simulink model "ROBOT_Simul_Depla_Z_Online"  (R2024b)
settings: Solver=ode15s  StartTime=0.0  StopTime=0.2  RelTol=1e-3  EnableMultiTasking=on
undefined symbols (not defined in the file): BATI1_Défaut_sldprt, BATI2_Défaut_sldprt, BATI3_Défaut_sldprt, BIELLE_Défaut_sldprt, BRAS_Défaut_sldprt, deg, Drive, EFFECTEUR_Défaut_sldprt, Fichiers, Fichiers_Matlab_sujetB, JOINT_Défaut_sldprt, kg, m, MANETTE_Défaut_sldprt, MATLAB, Matlab, mm, N, PIED_Défaut_sldprt, rad, s, STL, X, Y, Z
libraries: sm_lib x139, fl_lib x42, nesl_utility x19, slpidlib x3
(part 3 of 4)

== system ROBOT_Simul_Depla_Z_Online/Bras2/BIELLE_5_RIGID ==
  ReferenceFrame : sm_lib/Frames and Transforms/Reference Frame
  Solid : sm_lib/Body Elements/File Solid  ExtGeomFileName=/MATLAB Drive/Fichiers_Matlab_sujetB/Fichiers Matlab/STL/BIELLE_Défaut_sldprt.STL  UnitType=Custom  ExtGeomFileUnits=mm  StepReaderType=HEX  ExportConvexHullGeometry=off  InertiaType=Custom  BasedOnType=Density  Density=1000  DensityUnits=kg/(m^3)  Mass=0.008350539405564527  MassUnits=kg  CenterOfMass=[0 1.3968069938607398e-07 -5.4963035279888423e-06]  CenterOfMassUnits=mm  MomentsOfInertia=[9.7237898508136684 9.7147278737202658 0.035523108889582884]  MomentsOfInertiaUnits=kg*mm^2  ProductsOfInertia=[0 -4.4011490170351759e-08 -8.1673382975267321e-07]  ProductsOfInertiaUnits=kg*mm^2  GraphicType=FromGeometry  MarkerShape=Sphere  MarkerSize=10  GraphicVisPropType=SimpleVisualProperties  GraphicDiffuseColor=[0.69803921568627447 0.69803921568627447 0.69803921568627447]  GraphicOpacity=1  GraphicSpecularColor=[0.5 0.5 0.5 1.0]  GraphicAmbientColor=[0.15 0.15 0.15 1.0]  GraphicEmissiveColor=[0.0 0.0 0.0 1.0]  GraphicShininess=75  DoExposeReferenceFrame=on  SerializedFrames=<Frames/>
  Transform : sm_lib/Frames and Transforms/Rigid Transform  RotationMethod=ArbitraryAxis  FollAlignAxisA=+X  BaseAlignAxisA=+Y  FollAlignAxisB=+Y  BaseAlignAxisB=+Z  RotationStandardAxis=+Z  RotationAngle=2.0943951023931953  RotationAngleUnits=rad  RotationArbitraryAxis=[0.57735026918962584 -0.57735026918962584 0.57735026918962584]  RotationSequenceAxes=FollowerAxes  RotationSequence=XYX  RotationSequenceAngles=[0 0 0]  RotationSequenceAnglesUnits=deg  RotationMatrix=[1 0 0; 0 1 0; 0 0 1]  Quaternion=[1 0 0 0]  TranslationMethod=Cartesian  TranslationCartesianOffset=[0 4.9999999999999973 -51.250000000000007]  TranslationCartesianOffsetUnits=mm  TranslationStandardAxis=+Z  TranslationStandardOffset=0  TranslationStandardOffsetUnits=mm  TranslationROffset=0  TranslationROffsetUnits=m  TranslationThetaOffset=0  TranslationThetaOffsetUnits=deg  TranslationZOffset=0  TranslationZOffsetUnits=m
  Transform1 : sm_lib/Frames and Transforms/Rigid Transform  RotationMethod=ArbitraryAxis  FollAlignAxisA=+X  BaseAlignAxisA=+Y  FollAlignAxisB=+Y  BaseAlignAxisB=+Z  RotationStandardAxis=+Z  RotationAngle=2.0943951023931953  RotationAngleUnits=rad  RotationArbitraryAxis=[0.57735026918962584 -0.57735026918962584 0.57735026918962584]  RotationSequenceAxes=FollowerAxes  RotationSequence=XYX  RotationSequenceAngles=[0 0 0]  RotationSequenceAnglesUnits=deg  RotationMatrix=[1 0 0; 0 1 0; 0 0 1]  Quaternion=[1 0 0 0]  TranslationMethod=Cartesian  TranslationCartesianOffset=[0 5.0000000000000044 51.249999999999993]  TranslationCartesianOffsetUnits=mm  TranslationStandardAxis=+Z  TranslationStandardOffset=0  TranslationStandardOffsetUnits=mm  TranslationROffset=0  TranslationROffsetUnits=m  TranslationThetaOffset=0  TranslationThetaOffsetUnits=deg  TranslationZOffset=0  TranslationZOffsetUnits=m
  F : PMIOPort  Side=Left
  F1 : PMIOPort  Port=2  Side=Right
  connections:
  Solid/RConn1 -- ReferenceFrame/RConn1 -- Transform/LConn1 -- Transform1/LConn1
  Transform/RConn1 -- F/RConn1
  Transform1/RConn1 -- F1/RConn1

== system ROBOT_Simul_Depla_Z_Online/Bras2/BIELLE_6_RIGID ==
  ReferenceFrame : sm_lib/Frames and Transforms/Reference Frame
  Solid : sm_lib/Body Elements/File Solid  ExtGeomFileName=/MATLAB Drive/Fichiers_Matlab_sujetB/Fichiers Matlab/STL/BIELLE_Défaut_sldprt.STL  UnitType=Custom  ExtGeomFileUnits=mm  StepReaderType=HEX  ExportConvexHullGeometry=off  InertiaType=Custom  BasedOnType=Density  Density=1000  DensityUnits=kg/(m^3)  Mass=0.008350539405564527  MassUnits=kg  CenterOfMass=[0 1.3968069938607398e-07 -5.4963035279888423e-06]  CenterOfMassUnits=mm  MomentsOfInertia=[9.7237898508136684 9.7147278737202658 0.035523108889582884]  MomentsOfInertiaUnits=kg*mm^2  ProductsOfInertia=[0 -4.4011490170351759e-08 -8.1673382975267321e-07]  ProductsOfInertiaUnits=kg*mm^2  GraphicType=FromGeometry  MarkerShape=Sphere  MarkerSize=10  GraphicVisPropType=SimpleVisualProperties  GraphicDiffuseColor=[0.69803921568627447 0.69803921568627447 0.69803921568627447]  GraphicOpacity=1  GraphicSpecularColor=[0.5 0.5 0.5 1.0]  GraphicAmbientColor=[0.15 0.15 0.15 1.0]  GraphicEmissiveColor=[0.0 0.0 0.0 1.0]  GraphicShininess=75  DoExposeReferenceFrame=on  SerializedFrames=<Frames/>
  Transform : sm_lib/Frames and Transforms/Rigid Transform  RotationMethod=ArbitraryAxis  FollAlignAxisA=+X  BaseAlignAxisA=+Y  FollAlignAxisB=+Y  BaseAlignAxisB=+Z  RotationStandardAxis=+Z  RotationAngle=2.0943951023931953  RotationAngleUnits=rad  RotationArbitraryAxis=[0.57735026918962584 -0.57735026918962584 0.57735026918962584]  RotationSequenceAxes=FollowerAxes  RotationSequence=XYX  RotationSequenceAngles=[0 0 0]  RotationSequenceAnglesUnits=deg  RotationMatrix=[1 0 0; 0 1 0; 0 0 1]  Quaternion=[1 0 0 0]  TranslationMethod=Cartesian  TranslationCartesianOffset=[0 4.9999999999999902 -51.249999999999993]  TranslationCartesianOffsetUnits=mm  TranslationStandardAxis=+Z  TranslationStandardOffset=0  TranslationStandardOffsetUnits=mm  TranslationROffset=0  TranslationROffsetUnits=m  TranslationThetaOffset=0  TranslationThetaOffsetUnits=deg  TranslationZOffset=0  TranslationZOffsetUnits=m
  Transform1 : sm_lib/Frames and Transforms/Rigid Transform  RotationMethod=ArbitraryAxis  FollAlignAxisA=+X  BaseAlignAxisA=+Y  FollAlignAxisB=+Y  BaseAlignAxisB=+Z  RotationStandardAxis=+Z  RotationAngle=2.0943951023931953  RotationAngleUnits=rad  RotationArbitraryAxis=[0.57735026918962584 -0.57735026918962584 0.57735026918962584]  RotationSequenceAxes=FollowerAxes  RotationSequence=XYX  RotationSequenceAngles=[0 0 0]  RotationSequenceAnglesUnits=deg  RotationMatrix=[1 0 0; 0 1 0; 0 0 1]  Quaternion=[1 0 0 0]  TranslationMethod=Cartesian  TranslationCartesianOffset=[0 4.9999999999999902 51.25]  TranslationCartesianOffsetUnits=mm  TranslationStandardAxis=+Z  TranslationStandardOffset=0  TranslationStandardOffsetUnits=mm  TranslationROffset=0  TranslationROffsetUnits=m  TranslationThetaOffset=0  TranslationThetaOffsetUnits=deg  TranslationZOffset=0  TranslationZOffsetUnits=m
  F : PMIOPort  Side=Left
  F1 : PMIOPort  Port=2  Side=Right
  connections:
  Solid/RConn1 -- ReferenceFrame/RConn1 -- Transform/LConn1 -- Transform1/LConn1
  Transform/RConn1 -- F/RConn1
  Transform1/RConn1 -- F1/RConn1

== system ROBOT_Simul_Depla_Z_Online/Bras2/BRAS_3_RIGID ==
  BRAS_1_RIGID : Subsystem
  BRAS_3_RIGID : Subsystem
  ReferenceFrame : sm_lib/Frames and Transforms/Reference Frame
  Transform : sm_lib/Frames and Transforms/Rigid Transform  RotationMethod=ArbitraryAxis  FollAlignAxisA=+X  BaseAlignAxisA=+Y  FollAlignAxisB=+Y  BaseAlignAxisB=+Z  RotationStandardAxis=+Z  RotationAngle=3.1415926535897922  RotationAngleUnits=rad  RotationArbitraryAxis=[1 -3.4968219954323673e-31 -7.4654377952851924e-16]  RotationSequenceAxes=FollowerAxes  RotationSequence=XYX  RotationSequenceAngles=[0 0 0]  RotationSequenceAnglesUnits=deg  RotationMatrix=[1 0 0; 0 1 0; 0 0 1]  Quaternion=[1 0 0 0]  TranslationMethod=Cartesian  TranslationCartesianOffset=[-7.3896444519050419e-13 -16.842456388464797 5.0000000000063061]  TranslationCartesianOffsetUnits=mm  TranslationStandardAxis=+Z  TranslationStandardOffset=0  TranslationStandardOffsetUnits=mm  TranslationROffset=0  TranslationROffsetUnits=m  TranslationThetaOffset=0  TranslationThetaOffsetUnits=deg  TranslationZOffset=0  TranslationZOffsetUnits=m
  Transform1 : sm_lib/Frames and Transforms/Rigid Transform  RotationMethod=ArbitraryAxis  FollAlignAxisA=+X  BaseAlignAxisA=+Y  FollAlignAxisB=+Y  BaseAlignAxisB=+Z  RotationStandardAxis=+Z  RotationAngle=3.1415926535897931  RotationAngleUnits=rad  RotationArbitraryAxis=[1 0 0]  RotationSequenceAxes=FollowerAxes  RotationSequence=XYX  RotationSequenceAngles=[0 0 0]  RotationSequenceAnglesUnits=deg  RotationMatrix=[1 0 0; 0 1 0; 0 0 1]  Quaternion=[1 0 0 0]  TranslationMethod=Cartesian  TranslationCartesianOffset=[0 43.157543611535338 10.000000000006285]  TranslationCartesianOffsetUnits=mm  TranslationStandardAxis=+Z  TranslationStandardOffset=0  TranslationStandardOffsetUnits=mm  TranslationROffset=0  TranslationROffsetUnits=m  TranslationThetaOffset=0  TranslationThetaOffsetUnits=deg  TranslationZOffset=0  TranslationZOffsetUnits=m
  Transform2 : sm_lib/Frames and Transforms/Rigid Transform  RotationMethod=None  FollAlignAxisA=+X  BaseAlignAxisA=+Y  FollAlignAxisB=+Y  BaseAlignAxisB=+Z  RotationStandardAxis=+Z  RotationAngle=0  RotationAngleUnits=deg  RotationArbitraryAxis=[0 0 1]  RotationSequenceAxes=FollowerAxes  RotationSequence=XYX  RotationSequenceAngles=[0 0 0]  RotationSequenceAnglesUnits=deg  RotationMatrix=[1 0 0; 0 1 0; 0 0 1]  Quaternion=[1 0 0 0]  TranslationMethod=Cartesian  TranslationCartesianOffset=[0 -16.842456388464662 6.2762295360840881e-12]  TranslationCartesianOffsetUnits=mm  TranslationStandardAxis=+Z  TranslationStandardOffset=0  TranslationStandardOffsetUnits=mm  TranslationROffset=0  TranslationROffsetUnits=m  TranslationThetaOffset=0  TranslationThetaOffsetUnits=deg  TranslationZOffset=0  TranslationZOffsetUnits=m
  Transform3 : sm_lib/Frames and Transforms/Rigid Transform  RotationMethod=ArbitraryAxis  FollAlignAxisA=+X  BaseAlignAxisA=+Y  FollAlignAxisB=+Y  BaseAlignAxisB=+Z  RotationStandardAxis=+Z  RotationAngle=3.1415926535897931  RotationAngleUnits=rad  RotationArbitraryAxis=[0 0 1]  RotationSequenceAxes=FollowerAxes  RotationSequence=XYX  RotationSequenceAngles=[0 0 0]  RotationSequenceAnglesUnits=deg  RotationMatrix=[1 0 0; 0 1 0; 0 0 1]  Quaternion=[1 0 0 0]  TranslationMethod=Cartesian  TranslationCartesianOffset=[0 43.157543611535338 6.2692906421801808e-12]  TranslationCartesianOffsetUnits=mm  TranslationStandardAxis=+Z  TranslationStandardOffset=0  TranslationStandardOffsetUnits=mm  TranslationROffset=0  TranslationROffsetUnits=m  TranslationThetaOffset=0  TranslationThetaOffsetUnits=deg  TranslationZOffset=0  TranslationZOffsetUnits=m
  F : PMIOPort  Side=Left
  F1 : PMIOPort  Port=2  Side=Right
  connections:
  Transform/LConn1 -- ReferenceFrame/RConn1 -- Transform1/LConn1 -- Transform2/LConn1 -- Transform3/LConn1
  Transform/RConn1 -- F/RConn1
  Transform1/RConn1 -- F1/RConn1
  BRAS_1_RIGID/LConn1 -- Transform2/RConn1
  BRAS_3_RIGID/LConn1 -- Transform3/RConn1

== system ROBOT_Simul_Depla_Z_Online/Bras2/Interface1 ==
  Angular Velocity Source : fl_lib/Mechanical/Mechanical Sources/Ideal Angular Velocity Source
  Torque Sensor : fl_lib/Mechanical/Mechanical Sensors/Ideal Torque Sensor
  C : PMIOPort  Side=Left
  T : PMIOPort  Port=2  Side=Right
  w : PMIOPort  Port=3  Side=Right
  R : PMIOPort  Port=4  Side=Left
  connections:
  Angular Velocity Source/RConn1 -- w/RConn1
  C/RConn1 -- Torque Sensor/RConn1
  Torque Sensor/RConn2 -- T/RConn1
  Torque Sensor/LConn1 -- Angular Velocity Source/RConn2
  R/RConn1 -- Angular Velocity Source/LConn1

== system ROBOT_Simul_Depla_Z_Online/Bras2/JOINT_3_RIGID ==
  ReferenceFrame : sm_lib/Frames and Transforms/Reference Frame
  Solid : sm_lib/Body Elements/File Solid  ExtGeomFileName=/MATLAB Drive/Fichiers_Matlab_sujetB/Fichiers Matlab/STL/JOINT_Défaut_sldprt.STL  UnitType=Custom  ExtGeomFileUnits=mm  StepReaderType=HEX  ExportConvexHullGeometry=off  InertiaType=Custom  BasedOnType=Density  Density=1000  DensityUnits=kg/(m^3)  Mass=0.010425088409650831  MassUnits=kg  CenterOfMass=[-2.8413803884081348e-07 7.2198924235006832 8.2870434049836507e-08]  CenterOfMassUnits=mm  MomentsOfInertia=[0.40441054898779027 0.67355736496231777 0.88349580308055875]  MomentsOfInertiaUnits=kg*mm^2  ProductsOfInertia=[5.448486796310623e-10 1.7393207622030534e-07 1.1975376403711247e-08]  ProductsOfInertiaUnits=kg*mm^2  GraphicType=FromGeometry  MarkerShape=Sphere  MarkerSize=10  GraphicVisPropType=SimpleVisualProperties  GraphicDiffuseColor=[0.792156862745098 0.81960784313725488 0.93333333333333335]  GraphicOpacity=1  GraphicSpecularColor=[0.5 0.5 0.5 1.0]  GraphicAmbientColor=[0.15 0.15 0.15 1.0]  GraphicEmissiveColor=[0.0 0.0 0.0 1.0]  GraphicShininess=75  DoExposeReferenceFrame=on  SerializedFrames=<Frames/>
  Transform : sm_lib/Frames and Transforms/Rigid Transform  RotationMethod=ArbitraryAxis  FollAlignAxisA=+X  BaseAlignAxisA=+Y  FollAlignAxisB=+Y  BaseAlignAxisB=+Z  RotationStandardAxis=+Z  RotationAngle=3.1415926535897927  RotationAngleUnits=rad  RotationArbitraryAxis=[1 2.4716035461156956e-31 6.8614764825058098e-16]  RotationSequenceAxes=FollowerAxes  RotationSequence=XYX  RotationSequenceAngles=[0 0 0]  RotationSequenceAnglesUnits=deg  RotationMatrix=[1 0 0; 0 1 0; 0 0 1]  Quaternion=[1 0 0 0]  TranslationMethod=Cartesian  TranslationCartesianOffset=[14.000000000000393 5.0000000000002949 4.9999999999999307]  TranslationCartesianOffsetUnits=mm  TranslationStandardAxis=+Z  TranslationStandardOffset=0  TranslationStandardOffsetUnits=mm  TranslationROffset=0  TranslationROffsetUnits=m  TranslationThetaOffset=0  TranslationThetaOffsetUnits=deg  TranslationZOffset=0  TranslationZOffsetUnits=m
  Transform1 : sm_lib/Frames and Transforms/Rigid Transform  RotationMethod=ArbitraryAxis  FollAlignAxisA=+X  BaseAlignAxisA=+Y  FollAlignAxisB=+Y  BaseAlignAxisB=+Z  RotationStandardAxis=+Z  RotationAngle=3.1415926535897931  RotationAngleUnits=rad  RotationArbitraryAxis=[1 6.1605098685514057e-33 4.1234572726680469e-16]  RotationSequenceAxes=FollowerAxes  RotationSequence=XYX  RotationSequenceAngles=[0 0 0]  RotationSequenceAnglesUnits=deg  RotationMatrix=[1 0 0; 0 1 0; 0 0 1]  Quaternion=[1 0 0 0]  TranslationMethod=Cartesian  TranslationCartesianOffset=[-13.999999999999581 5.0000000000001972 4.9999999999999769]  TranslationCartesianOffsetUnits=mm  TranslationStandardAxis=+Z  TranslationStandardOffset=0  TranslationStandardOffsetUnits=mm  TranslationROffset=0  TranslationROffsetUnits=m  TranslationThetaOffset=0  TranslationThetaOffsetUnits=deg  TranslationZOffset=0  TranslationZOffsetUnits=m
  Transform2 : sm_lib/Frames and Transforms/Rigid Transform  RotationMethod=ArbitraryAxis  FollAlignAxisA=+X  BaseAlignAxisA=+Y  FollAlignAxisB=+Y  BaseAlignAxisB=+Z  RotationStandardAxis=+Z  RotationAngle=2.0943951023931962  RotationAngleUnits=rad  RotationArbitraryAxis=[0.57735026918962506 0.57735026918962606 0.57735026918962606]  RotationSequenceAxes=FollowerAxes  RotationSequence=XYX  RotationSequenceAngles=[0 0 0]  RotationSequenceAnglesUnits=deg  RotationMatrix=[1 0 0; 0 1 0; 0 0 1]  Quaternion=[1 0 0 0]  TranslationMethod=Cartesian  TranslationCartesianOffset=[-10.000000000000021 16.250000000001698 1.8616219676914625e-12]  TranslationCartesianOffsetUnits=mm  TranslationStandardAxis=+Z  TranslationStandardOffset=0  TranslationStandardOffsetUnits=mm  TranslationROffset=0  TranslationROffsetUnits=m  TranslationThetaOffset=0  TranslationThetaOffsetUnits=deg  TranslationZOffset=0  TranslationZOffsetUnits=m
  F2 : PMIOPort  Side=Left
  F1 : PMIOPort  Port=2  Side=Right
  F : PMIOPort  Port=3  Side=Right
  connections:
  Solid/RConn1 -- ReferenceFrame/RConn1 -- Transform1/LConn1 -- Transform2/LConn1 -- Transform/LConn1
  Transform/RConn1 -- F/RConn1
  Transform1/RConn1 -- F1/RConn1
  Transform2/RConn1 -- F2/RConn1

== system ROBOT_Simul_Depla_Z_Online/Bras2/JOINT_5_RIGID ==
  ReferenceFrame : sm_lib/Frames and Transforms/Reference Frame
  Solid : sm_lib/Body Elements/File Solid  ExtGeomFileName=/MATLAB Drive/Fichiers_Matlab_sujetB/Fichiers Matlab/STL/JOINT_Défaut_sldprt.STL  UnitType=Custom  ExtGeomFileUnits=mm  StepReaderType=HEX  ExportConvexHullGeometry=off  InertiaType=Custom  BasedOnType=Density  Density=1000  DensityUnits=kg/(m^3)  Mass=0.010425088409650831  MassUnits=kg  CenterOfMass=[-2.8413803884081348e-07 7.2198924235006832 8.2870434049836507e-08]  CenterOfMassUnits=mm  MomentsOfInertia=[0.40441054898779027 0.67355736496231777 0.88349580308055875]  MomentsOfInertiaUnits=kg*mm^2  ProductsOfInertia=[5.448486796310623e-10 1.7393207622030534e-07 1.1975376403711247e-08]  ProductsOfInertiaUnits=kg*mm^2  GraphicType=FromGeometry  MarkerShape=Sphere  MarkerSize=10  GraphicVisPropType=SimpleVisualProperties  GraphicDiffuseColor=[0.792156862745098 0.81960784313725488 0.93333333333333335]  GraphicOpacity=1  GraphicSpecularColor=[0.5 0.5 0.5 1.0]  GraphicAmbientColor=[0.15 0.15 0.15 1.0]  GraphicEmissiveColor=[0.0 0.0 0.0 1.0]  GraphicShininess=75  DoExposeReferenceFrame=on  SerializedFrames=<Frames/>
  Transform : sm_lib/Frames and Transforms/Rigid Transform  RotationMethod=ArbitraryAxis  FollAlignAxisA=+X  BaseAlignAxisA=+Y  FollAlignAxisB=+Y  BaseAlignAxisB=+Z  RotationStandardAxis=+Z  RotationAngle=3.1415926535897931  RotationAngleUnits=rad  RotationArbitraryAxis=[-1 -6.4240613722994368e-33 4.1034435102868363e-17]  RotationSequenceAxes=FollowerAxes  RotationSequence=XYX  RotationSequenceAngles=[0 0 0]  RotationSequenceAnglesUnits=deg  RotationMatrix=[1 0 0; 0 1 0; 0 0 1]  Quaternion=[1 0 0 0]  TranslationMethod=Cartesian  TranslationCartesianOffset=[-13.99999999999973 4.9999999999999307 4.9999999999999662]  TranslationCartesianOffsetUnits=mm  TranslationStandardAxis=+Z  TranslationStandardOffset=0  TranslationStandardOffsetUnits=mm  TranslationROffset=0  TranslationROffsetUnits=m  TranslationThetaOffset=0  TranslationThetaOffsetUnits=deg  TranslationZOffset=0  TranslationZOffsetUnits=m
  Transform1 : sm_lib/Frames and Transforms/Rigid Transform  RotationMethod=ArbitraryAxis  FollAlignAxisA=+X  BaseAlignAxisA=+Y  FollAlignAxisB=+Y  BaseAlignAxisB=+Z  RotationStandardAxis=+Z  RotationAngle=3.1415926535897927  RotationAngleUnits=rad  RotationArbitraryAxis=[1 5.1356244409297584e-32 2.9638105957297091e-16]  RotationSequenceAxes=FollowerAxes  RotationSequence=XYX  RotationSequenceAngles=[0 0 0]  RotationSequenceAnglesUnits=deg  RotationMatrix=[1 0 0; 0 1 0; 0 0 1]  Quaternion=[1 0 0 0]  TranslationMethod=Cartesian  TranslationCartesianOffset=[14.000000000000249 4.9999999999997691 4.9999999999999734]  TranslationCartesianOffsetUnits=mm  TranslationStandardAxis=+Z  TranslationStandardOffset=0  TranslationStandardOffsetUnits=mm  TranslationROffset=0  TranslationROffsetUnits=m  TranslationThetaOffset=0  TranslationThetaOffsetUnits=deg  TranslationZOffset=0  TranslationZOffsetUnits=m
  Transform2 : sm_lib/Frames and Transforms/Rigid Transform  RotationMethod=ArbitraryAxis  FollAlignAxisA=+X  BaseAlignAxisA=+Y  FollAlignAxisB=+Y  BaseAlignAxisB=+Z  RotationStandardAxis=+Z  RotationAngle=2.0943951023931962  RotationAngleUnits=rad  RotationArbitraryAxis=[-0.57735026918962651 -0.57735026918962606 0.57735026918962473]  RotationSequenceAxes=FollowerAxes  RotationSequence=XYX  RotationSequenceAngles=[0 0 0]  RotationSequenceAnglesUnits=deg  RotationMatrix=[1 0 0; 0 1 0; 0 0 1]  Quaternion=[1 0 0 0]  TranslationMethod=Cartesian  TranslationCartesianOffset=[10.000000000000179 16.249999999999421 -3.836930773104541e-13]  TranslationCartesianOffsetUnits=mm  TranslationStandardAxis=+Z  TranslationStandardOffset=0  TranslationStandardOffsetUnits=mm  TranslationROffset=0  TranslationROffsetUnits=m  TranslationThetaOffset=0  TranslationThetaOffsetUnits=deg  TranslationZOffset=0  TranslationZOffsetUnits=m
  F1 : PMIOPort  Side=Left
  F : PMIOPort  Port=2  Side=Left
  F2 : PMIOPort  Port=3  Side=Right
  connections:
  Solid/RConn1 -- ReferenceFrame/RConn1 -- Transform1/LConn1 -- Transform2/LConn1 -- Transform/LConn1
  Transform/RConn1 -- F/RConn1
  Transform1/RConn1 -- F1/RConn1
  Transform2/RConn1 -- F2/RConn1

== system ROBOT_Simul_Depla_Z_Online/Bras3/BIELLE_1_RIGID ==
  ReferenceFrame : sm_lib/Frames and Transforms/Reference Frame
  Solid : sm_lib/Body Elements/File Solid  ExtGeomFileName=/MATLAB Drive/Fichiers_Matlab_sujetB/Fichiers Matlab/STL/BIELLE_Défaut_sldprt.STL  UnitType=Custom  ExtGeomFileUnits=mm  StepReaderType=HEX  ExportConvexHullGeometry=off  InertiaType=Custom  BasedOnType=Density  Density=1000  DensityUnits=kg/(m^3)  Mass=0.008350539405564527  MassUnits=kg  CenterOfMass=[0 1.3968069938607398e-07 -5.4963035279888423e-06]  CenterOfMassUnits=mm  MomentsOfInertia=[9.7237898508136684 9.7147278737202658 0.035523108889582884]  MomentsOfInertiaUnits=kg*mm^2  ProductsOfInertia=[0 -4.4011490170351759e-08 -8.1673382975267321e-07]  ProductsOfInertiaUnits=kg*mm^2  GraphicType=FromGeometry  MarkerShape=Sphere  MarkerSize=10  GraphicVisPropType=SimpleVisualProperties  GraphicDiffuseColor=[0.69803921568627447 0.69803921568627447 0.69803921568627447]  GraphicOpacity=1  GraphicSpecularColor=[0.5 0.5 0.5 1.0]  GraphicAmbientColor=[0.15 0.15 0.15 1.0]  GraphicEmissiveColor=[0.0 0.0 0.0 1.0]  GraphicShininess=75  DoExposeReferenceFrame=on  SerializedFrames=<Frames/>
  Transform : sm_lib/Frames and Transforms/Rigid Transform  RotationMethod=ArbitraryAxis  FollAlignAxisA=+X  BaseAlignAxisA=+Y  FollAlignAxisB=+Y  BaseAlignAxisB=+Z  RotationStandardAxis=+Z  RotationAngle=2.0943951023931953  RotationAngleUnits=rad  RotationArbitraryAxis=[-0.57735026918962584 -0.57735026918962584 -0.57735026918962584]  RotationSequenceAxes=FollowerAxes  RotationSequence=XYX  RotationSequenceAngles=[0 0 0]  RotationSequenceAnglesUnits=deg  RotationMatrix=[1 0 0; 0 1 0; 0 0 1]  Quaternion=[1 0 0 0]  TranslationMethod=Cartesian  TranslationCartesianOffset=[6.4659388954169117e-13 -4.9999999999998401 -51.250000000000263]  TranslationCartesianOffsetUnits=mm  TranslationStandardAxis=+Z  TranslationStandardOffset=0  TranslationStandardOffsetUnits=mm  TranslationROffset=0  TranslationROffsetUnits=m  TranslationThetaOffset=0  TranslationThetaOffsetUnits=deg  TranslationZOffset=0  TranslationZOffsetUnits=m
  Transform1 : sm_lib/Frames and Transforms/Rigid Transform  RotationMethod=ArbitraryAxis  FollAlignAxisA=+X  BaseAlignAxisA=+Y  FollAlignAxisB=+Y  BaseAlignAxisB=+Z  RotationStandardAxis=+Z  RotationAngle=2.0943951023931953  RotationAngleUnits=rad  RotationArbitraryAxis=[0.57735026918962584 -0.57735026918962584 0.57735026918962584]  RotationSequenceAxes=FollowerAxes  RotationSequence=XYX  RotationSequenceAngles=[0 0 0]  RotationSequenceAnglesUnits=deg  RotationMatrix=[1 0 0; 0 1 0; 0 0 1]  Quaternion=[1 0 0 0]  TranslationMethod=Cartesian  TranslationCartesianOffset=[0 4.9999999999999973 51.249999999999986]  TranslationCartesianOffsetUnits=mm  TranslationStandardAxis=+Z  TranslationStandardOffset=0  TranslationStandardOffsetUnits=mm  TranslationROffset=0  TranslationROffsetUnits=m  TranslationThetaOffset=0  TranslationThetaOffsetUnits=deg  TranslationZOffset=0  TranslationZOffsetUnits=m
  F : PMIOPort  Side=Left
  F1 : PMIOPort  Port=2  Side=Right
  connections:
  Solid/RConn1 -- ReferenceFrame/RConn1 -- Transform/LConn1 -- Transform1/LConn1
  Transform/RConn1 -- F/RConn1
  Transform1/RConn1 -- F1/RConn1

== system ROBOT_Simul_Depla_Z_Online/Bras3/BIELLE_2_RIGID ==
  ReferenceFrame : sm_lib/Frames and Transforms/Reference Frame
  Solid : sm_lib/Body Elements/File Solid  ExtGeomFileName=/MATLAB Drive/Fichiers_Matlab_sujetB/Fichiers Matlab/STL/BIELLE_Défaut_sldprt.STL  UnitType=Custom  ExtGeomFileUnits=mm  StepReaderType=HEX  ExportConvexHullGeometry=off  InertiaType=Custom  BasedOnType=Density  Density=1000  DensityUnits=kg/(m^3)  Mass=0.008350539405564527  MassUnits=kg  CenterOfMass=[0 1.3968069938607398e-07 -5.4963035279888423e-06]  CenterOfMassUnits=mm  MomentsOfInertia=[9.7237898508136684 9.7147278737202658 0.035523108889582884]  MomentsOfInertiaUnits=kg*mm^2  ProductsOfInertia=[0 -4.4011490170351759e-08 -8.1673382975267321e-07]  ProductsOfInertiaUnits=kg*mm^2  GraphicType=FromGeometry  MarkerShape=Sphere  MarkerSize=10  GraphicVisPropType=SimpleVisualProperties  GraphicDiffuseColor=[0.69803921568627447 0.69803921568627447 0.69803921568627447]  GraphicOpacity=1  GraphicSpecularColor=[0.5 0.5 0.5 1.0]  GraphicAmbientColor=[0.15 0.15 0.15 1.0]  GraphicEmissiveColor=[0.0 0.0 0.0 1.0]  GraphicShininess=75  DoExposeReferenceFrame=on  SerializedFrames=<Frames/>
  Transform : sm_lib/Frames and Transforms/Rigid Transform  RotationMethod=ArbitraryAxis  FollAlignAxisA=+X  BaseAlignAxisA=+Y  FollAlignAxisB=+Y  BaseAlignAxisB=+Z  RotationStandardAxis=+Z  RotationAngle=2.0943951023931944  RotationAngleUnits=rad  RotationArbitraryAxis=[-0.5773502691896254 -0.57735026918962551 -0.5773502691896264]  RotationSequenceAxes=FollowerAxes  RotationSequence=XYX  RotationSequenceAngles=[0 0 0]  RotationSequenceAnglesUnits=deg  RotationMatrix=[1 0 0; 0 1 0; 0 0 1]  Quaternion=[1 0 0 0]  TranslationMethod=Cartesian  TranslationCartesianOffset=[-6.5369931689929217e-13 -5.0000000000000746 51.250000000000604]  TranslationCartesianOffsetUnits=mm  TranslationStandardAxis=+Z  TranslationStandardOffset=0  TranslationStandardOffsetUnits=mm  TranslationROffset=0  TranslationROffsetUnits=m  TranslationThetaOffset=0  TranslationThetaOffsetUnits=deg  TranslationZOffset=0  TranslationZOffsetUnits=m
  Transform1 : sm_lib/Frames and Transforms/Rigid Transform  RotationMethod=ArbitraryAxis  FollAlignAxisA=+X  BaseAlignAxisA=+Y  FollAlignAxisB=+Y  BaseAlignAxisB=+Z  RotationStandardAxis=+Z  RotationAngle=2.0943951023931953  RotationAngleUnits=rad  RotationArbitraryAxis=[0.57735026918962584 -0.57735026918962584 0.57735026918962584]  RotationSequenceAxes=FollowerAxes  RotationSequence=XYX  RotationSequenceAngles=[0 0 0]  RotationSequenceAnglesUnits=deg  RotationMatrix=[1 0 0; 0 1 0; 0 0 1]  Quaternion=[1 0 0 0]  TranslationMethod=Cartesian  TranslationCartesianOffset=[0 4.9999999999999902 -51.250000000000007]  TranslationCartesianOffsetUnits=mm  TranslationStandardAxis=+Z  TranslationStandardOffset=0  TranslationStandardOffsetUnits=mm  TranslationROffset=0  TranslationROffsetUnits=m  TranslationThetaOffset=0  TranslationThetaOffsetUnits=deg  TranslationZOffset=0  TranslationZOffsetUnits=m
  F : PMIOPort  Side=Left
  F1 : PMIOPort  Port=2  Side=Right
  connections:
  Solid/RConn1 -- ReferenceFrame/RConn1 -- Transform/LConn1 -- Transform1/LConn1
  Transform/RConn1 -- F/RConn1
  Transform1/RConn1 -- F1/RConn1

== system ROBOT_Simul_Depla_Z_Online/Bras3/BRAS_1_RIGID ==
  BRAS_1_RIGID : Subsystem
  BRAS_3_RIGID : Subsystem
  ReferenceFrame : sm_lib/Frames and Transforms/Reference Frame
  Transform : sm_lib/Frames and Transforms/Rigid Transform  RotationMethod=ArbitraryAxis  FollAlignAxisA=+X  BaseAlignAxisA=+Y  FollAlignAxisB=+Y  BaseAlignAxisB=+Z  RotationStandardAxis=+Z  RotationAngle=3.1415926535897931  RotationAngleUnits=rad  RotationArbitraryAxis=[1 0 -1.0717459516511952e-16]  RotationSequenceAxes=FollowerAxes  RotationSequence=XYX  RotationSequenceAngles=[0 0 0]  RotationSequenceAnglesUnits=deg  RotationMatrix=[1 0 0; 0 1 0; 0 0 1]  Quaternion=[1 0 0 0]  TranslationMethod=Cartesian  TranslationCartesianOffset=[0 -16.842456388464662 10.000000000006278]  TranslationCartesianOffsetUnits=mm  TranslationStandardAxis=+Z  TranslationStandardOffset=0  TranslationStandardOffsetUnits=mm  TranslationROffset=0  TranslationROffsetUnits=m  TranslationThetaOffset=0  TranslationThetaOffsetUnits=deg  TranslationZOffset=0  TranslationZOffsetUnits=m
  Transform1 : sm_lib/Frames and Transforms/Rigid Transform  RotationMethod=ArbitraryAxis  FollAlignAxisA=+X  BaseAlignAxisA=+Y  FollAlignAxisB=+Y  BaseAlignAxisB=+Z  RotationStandardAxis=+Z  RotationAngle=3.1415926535897931  RotationAngleUnits=rad  RotationArbitraryAxis=[1 0 8.2888466501444268e-17]  RotationSequenceAxes=FollowerAxes  RotationSequence=XYX  RotationSequenceAngles=[0 0 0]  RotationSequenceAnglesUnits=deg  RotationMatrix=[1 0 0; 0 1 0; 0 0 1]  Quaternion=[1 0 0 0]  TranslationMethod=Cartesian  TranslationCartesianOffset=[-1.6577693300288846e-15 43.157543611535331 10.000000000006278]  TranslationCartesianOffsetUnits=mm  TranslationStandardAxis=+Z  TranslationStandardOffset=0  TranslationStandardOffsetUnits=mm  TranslationROffset=0  TranslationROffsetUnits=m  TranslationThetaOffset=0  TranslationThetaOffsetUnits=deg  TranslationZOffset=0  TranslationZOffsetUnits=m
  Transform2 : sm_lib/Frames and Transforms/Rigid Transform  RotationMethod=None  FollAlignAxisA=+X  BaseAlignAxisA=+Y  FollAlignAxisB=+Y  BaseAlignAxisB=+Z  RotationStandardAxis=+Z  RotationAngle=0  RotationAngleUnits=deg  RotationArbitraryAxis=[0 0 1]  RotationSequenceAxes=FollowerAxes  RotationSequence=XYX  RotationSequenceAngles=[0 0 0]  RotationSequenceAnglesUnits=deg  RotationMatrix=[1 0 0; 0 1 0; 0 0 1]  Quaternion=[1 0 0 0]  TranslationMethod=Cartesian  TranslationCartesianOffset=[0 -16.842456388464662 6.2727600891321345e-12]  TranslationCartesianOffsetUnits=mm  TranslationStandardAxis=+Z  TranslationStandardOffset=0  TranslationStandardOffsetUnits=mm  TranslationROffset=0  TranslationROffsetUnits=m  TranslationThetaOffset=0  TranslationThetaOffsetUnits=deg  TranslationZOffset=0  TranslationZOffsetUnits=m
  Transform3 : sm_lib/Frames and Transforms/Rigid Transform  RotationMethod=ArbitraryAxis  FollAlignAxisA=+X  BaseAlignAxisA=+Y  FollAlignAxisB=+Y  BaseAlignAxisB=+Z  RotationStandardAxis=+Z  RotationAngle=3.1415926535897931  RotationAngleUnits=rad  RotationArbitraryAxis=[-8.2888466501444268e-17 0 1]  RotationSequenceAxes=FollowerAxes  RotationSequence=XYX  RotationSequenceAngles=[0 0 0]  RotationSequenceAnglesUnits=deg  RotationMatrix=[1 0 0; 0 1 0; 0 0 1]  Quaternion=[1 0 0 0]  TranslationMethod=Cartesian  TranslationCartesianOffset=[0 43.157543611535331 6.2831684299879953e-12]  TranslationCartesianOffsetUnits=mm  TranslationStandardAxis=+Z  TranslationStandardOffset=0  TranslationStandardOffsetUnits=mm  TranslationROffset=0  TranslationROffsetUnits=m  TranslationThetaOffset=0  TranslationThetaOffsetUnits=deg  TranslationZOffset=0  TranslationZOffsetUnits=m
  F1 : PMIOPort  Side=Right
  F : PMIOPort  Port=2  Side=Left
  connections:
  Transform/LConn1 -- ReferenceFrame/RConn1 -- Transform1/LConn1 -- Transform2/LConn1 -- Transform3/LConn1
  Transform/RConn1 -- F/RConn1
  Transform1/RConn1 -- F1/RConn1
  BRAS_1_RIGID/LConn1 -- Transform2/RConn1
  BRAS_3_RIGID/LConn1 -- Transform3/RConn1

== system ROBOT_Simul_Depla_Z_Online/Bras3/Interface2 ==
  Angular Velocity Source : fl_lib/Mechanical/Mechanical Sources/Ideal Angular Velocity Source
  Torque Sensor : fl_lib/Mechanical/Mechanical Sensors/Ideal Torque Sensor
  C : PMIOPort  Side=Left
  T : PMIOPort  Port=2  Side=Right
  w : PMIOPort  Port=3  Side=Right
  R : PMIOPort  Port=4  Side=Left
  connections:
  R/RConn1 -- Angular Velocity Source/LConn1
  Torque Sensor/LConn1 -- Angular Velocity Source/RConn2
  Torque Sensor/RConn2 -- T/RConn1
  C/RConn1 -- Torque Sensor/RConn1
  Angular Velocity Source/RConn1 -- w/RConn1

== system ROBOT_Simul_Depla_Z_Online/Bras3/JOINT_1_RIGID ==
  ReferenceFrame : sm_lib/Frames and Transforms/Reference Frame
  Solid : sm_lib/Body Elements/File Solid  ExtGeomFileName=/MATLAB Drive/Fichiers_Matlab_sujetB/Fichiers Matlab/STL/JOINT_Défaut_sldprt.STL  UnitType=Custom  ExtGeomFileUnits=mm  StepReaderType=HEX  ExportConvexHullGeometry=off  InertiaType=Custom  BasedOnType=Density  Density=1000  DensityUnits=kg/(m^3)  Mass=0.010425088409650831  MassUnits=kg  CenterOfMass=[-2.8413803884081348e-07 7.2198924235006832 8.2870434049836507e-08]  CenterOfMassUnits=mm  MomentsOfInertia=[0.40441054898779027 0.67355736496231777 0.88349580308055875]  MomentsOfInertiaUnits=kg*mm^2  ProductsOfInertia=[5.448486796310623e-10 1.7393207622030534e-07 1.1975376403711247e-08]  ProductsOfInertiaUnits=kg*mm^2  GraphicType=FromGeometry  MarkerShape=Sphere  MarkerSize=10  GraphicVisPropType=SimpleVisualProperties  GraphicDiffuseColor=[0.792156862745098 0.81960784313725488 0.93333333333333335]  GraphicOpacity=1  GraphicSpecularColor=[0.5 0.5 0.5 1.0]  GraphicAmbientColor=[0.15 0.15 0.15 1.0]  GraphicEmissiveColor=[0.0 0.0 0.0 1.0]  GraphicShininess=75  DoExposeReferenceFrame=on  SerializedFrames=<Frames/>
  Transform : sm_lib/Frames and Transforms/Rigid Transform  RotationMethod=ArbitraryAxis  FollAlignAxisA=+X  BaseAlignAxisA=+Y  FollAlignAxisB=+Y  BaseAlignAxisB=+Z  RotationStandardAxis=+Z  RotationAngle=3.1415926535897931  RotationAngleUnits=rad  RotationArbitraryAxis=[1 0 -5.6857825516938873e-17]  RotationSequenceAxes=FollowerAxes  RotationSequence=XYX  RotationSequenceAngles=[0 0 0]  RotationSequenceAnglesUnits=deg  RotationMatrix=[1 0 0; 0 1 0; 0 0 1]  Quaternion=[1 0 0 0]  TranslationMethod=Cartesian  TranslationCartesianOffset=[-13.999999999999998 5.0000000000000115 5.0000000000000187]  TranslationCartesianOffsetUnits=mm  TranslationStandardAxis=+Z  TranslationStandardOffset=0  TranslationStandardOffsetUnits=mm  TranslationROffset=0  TranslationROffsetUnits=m  TranslationThetaOffset=0  TranslationThetaOffsetUnits=deg  TranslationZOffset=0  TranslationZOffsetUnits=m
  Transform1 : sm_lib/Frames and Transforms/Rigid Transform  RotationMethod=ArbitraryAxis  FollAlignAxisA=+X  BaseAlignAxisA=+Y  FollAlignAxisB=+Y  BaseAlignAxisB=+Z  RotationStandardAxis=+Z  RotationAngle=3.1415926535897931  RotationAngleUnits=rad  RotationArbitraryAxis=[1 0 -5.6857825516938873e-17]  RotationSequenceAxes=FollowerAxes  RotationSequence=XYX  RotationSequenceAngles=[0 0 0]  RotationSequenceAnglesUnits=deg  RotationMatrix=[1 0 0; 0 1 0; 0 0 1]  Quaternion=[1 0 0 0]  TranslationMethod=Cartesian  TranslationCartesianOffset=[14.000000000000009 4.9999999999999973 5.0000000000000044]  TranslationCartesianOffsetUnits=mm  TranslationStandardAxis=+Z  TranslationStandardOffset=0  TranslationStandardOffsetUnits=mm  TranslationROffset=0  TranslationROffsetUnits=m  TranslationThetaOffset=0  TranslationThetaOffsetUnits=deg  TranslationZOffset=0  TranslationZOffsetUnits=m
  Transform2 : sm_lib/Frames and Transforms/Rigid Transform  RotationMethod=ArbitraryAxis  FollAlignAxisA=+X  BaseAlignAxisA=+Y  FollAlignAxisB=+Y  BaseAlignAxisB=+Z  RotationStandardAxis=+Z  RotationAngle=2.0943951023931953  RotationAngleUnits=rad  RotationArbitraryAxis=[-0.57735026918962584 -0.57735026918962562 0.57735026918962595]  RotationSequenceAxes=FollowerAxes  RotationSequence=XYX  RotationSequenceAngles=[0 0 0]  RotationSequenceAnglesUnits=deg  RotationMatrix=[1 0 0; 0 1 0; 0 0 1]  Quaternion=[1 0 0 0]  TranslationMethod=Cartesian  TranslationCartesianOffset=[10.000000000006255 16.249999999999446 5.3290705182007514e-13]  TranslationCartesianOffsetUnits=mm  TranslationStandardAxis=+Z  TranslationStandardOffset=0  TranslationStandardOffsetUnits=mm  TranslationROffset=0  TranslationROffsetUnits=m  TranslationThetaOffset=0  TranslationThetaOffsetUnits=deg  TranslationZOffset=0  TranslationZOffsetUnits=m
  F2 : PMIOPort  Side=Left
  F1 : PMIOPort  Port=2  Side=Right
  F : PMIOPort  Port=3  Side=Right
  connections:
  Solid/RConn1 -- ReferenceFrame/RConn1 -- Transform1/LConn1 -- Transform2/LConn1 -- Transform/LConn1
  Transform/RConn1 -- F/RConn1
  Transform1/RConn1 -- F1/RConn1
  Transform2/RConn1 -- F2/RConn1

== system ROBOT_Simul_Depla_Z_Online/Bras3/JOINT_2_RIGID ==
  ReferenceFrame : sm_lib/Frames and Transforms/Reference Frame
  Solid : sm_lib/Body Elements/File Solid  ExtGeomFileName=/MATLAB Drive/Fichiers_Matlab_sujetB/Fichiers Matlab/STL/JOINT_Défaut_sldprt.STL  UnitType=Custom  ExtGeomFileUnits=mm  StepReaderType=HEX  ExportConvexHullGeometry=off  InertiaType=Custom  BasedOnType=Density  Density=1000  DensityUnits=kg/(m^3)  Mass=0.010425088409650831  MassUnits=kg  CenterOfMass=[-2.8413803884081348e-07 7.2198924235006832 8.2870434049836507e-08]  CenterOfMassUnits=mm  MomentsOfInertia=[0.40441054898779027 0.67355736496231777 0.88349580308055875]  MomentsOfInertiaUnits=kg*mm^2  ProductsOfInertia=[5.448486796310623e-10 1.7393207622030534e-07 1.1975376403711247e-08]  ProductsOfInertiaUnits=kg*mm^2  GraphicType=FromGeometry  MarkerShape=Sphere  MarkerSize=10  GraphicVisPropType=SimpleVisualProperties  GraphicDiffuseColor=[0.792156862745098 0.81960784313725488 0.93333333333333335]  GraphicOpacity=1  GraphicSpecularColor=[0.5 0.5 0.5 1.0]  GraphicAmbientColor=[0.15 0.15 0.15 1.0]  GraphicEmissiveColor=[0.0 0.0 0.0 1.0]  GraphicShininess=75  DoExposeReferenceFrame=on  SerializedFrames=<Frames/>
  Transform : sm_lib/Frames and Transforms/Rigid Transform  RotationMethod=ArbitraryAxis  FollAlignAxisA=+X  BaseAlignAxisA=+Y  FollAlignAxisB=+Y  BaseAlignAxisB=+Z  RotationStandardAxis=+Z  RotationAngle=3.1415926535897931  RotationAngleUnits=rad  RotationArbitraryAxis=[1 1.6269902822629644e-32 1.2901180678782253e-16]  RotationSequenceAxes=FollowerAxes  RotationSequence=XYX  RotationSequenceAngles=[0 0 0]  RotationSequenceAnglesUnits=deg  RotationMatrix=[1 0 0; 0 1 0; 0 0 1]  Quaternion=[1 0 0 0]  TranslationMethod=Cartesian  TranslationCartesianOffset=[-13.999999999999371 4.9999999999998597 4.9999999999998881]  TranslationCartesianOffsetUnits=mm  TranslationStandardAxis=+Z  TranslationStandardOffset=0  TranslationStandardOffsetUnits=mm  TranslationROffset=0  TranslationROffsetUnits=m  TranslationThetaOffset=0  TranslationThetaOffsetUnits=deg  TranslationZOffset=0  TranslationZOffsetUnits=m
  Transform1 : sm_lib/Frames and Transforms/Rigid Transform  RotationMethod=ArbitraryAxis  FollAlignAxisA=+X  BaseAlignAxisA=+Y  FollAlignAxisB=+Y  BaseAlignAxisB=+Z  RotationStandardAxis=+Z  RotationAngle=3.1415926535897909  RotationAngleUnits=rad  RotationArbitraryAxis=[1 -3.616260618277222e-32 -3.0826822740225111e-17]  RotationSequenceAxes=FollowerAxes  RotationSequence=XYX  RotationSequenceAngles=[0 0 0]  RotationSequenceAnglesUnits=deg  RotationMatrix=[1 0 0; 0 1 0; 0 0 1]  Quaternion=[1 0 0 0]  TranslationMethod=Cartesian  TranslationCartesianOffset=[14.000000000000639 5.0000000000006715 4.9999999999999156]  TranslationCartesianOffsetUnits=mm  TranslationStandardAxis=+Z  TranslationStandardOffset=0  TranslationStandardOffsetUnits=mm  TranslationROffset=0  TranslationROffsetUnits=m  TranslationThetaOffset=0  TranslationThetaOffsetUnits=deg  TranslationZOffset=0  TranslationZOffsetUnits=m
  Transform2 : sm_lib/Frames and Transforms/Rigid Transform  RotationMethod=ArbitraryAxis  FollAlignAxisA=+X  BaseAlignAxisA=+Y  FollAlignAxisB=+Y  BaseAlignAxisB=+Z  RotationStandardAxis=+Z  RotationAngle=2.0943951023931953  RotationAngleUnits=rad  RotationArbitraryAxis=[-0.57735026918962584 -0.57735026918962584 0.57735026918962584]  RotationSequenceAxes=FollowerAxes  RotationSequence=XYX  RotationSequenceAngles=[0 0 0]  RotationSequenceAnglesUnits=deg  RotationMatrix=[1 0 0; 0 1 0; 0 0 1]  Quaternion=[1 0 0 0]  TranslationMethod=Cartesian  TranslationCartesianOffset=[4.9999999999999973 16.249999999999993 0]  TranslationCartesianOffsetUnits=mm  TranslationStandardAxis=+Z  TranslationStandardOffset=0  TranslationStandardOffsetUnits=mm  TranslationROffset=0  TranslationROffsetUnits=m  TranslationThetaOffset=0  TranslationThetaOffsetUnits=deg  TranslationZOffset=0  TranslationZOffsetUnits=m
  F1 : PMIOPort  Side=Left
  F : PMIOPort  Port=2  Side=Left
  F2 : PMIOPort  Port=3  Side=Right
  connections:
  Solid/RConn1 -- ReferenceFrame/RConn1 -- Transform1/LConn1 -- Transform2/LConn1 -- Transform/LConn1
  Transform/RConn1 -- F/RConn1
  Transform1/RConn1 -- F1/RConn1
  Transform2/RConn1 -- F2/RConn1

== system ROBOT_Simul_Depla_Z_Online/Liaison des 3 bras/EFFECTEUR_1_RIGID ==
  ReferenceFrame : sm_lib/Frames and Transforms/Reference Frame
  Solid : sm_lib/Body Elements/File Solid  ExtGeomFileName=/MATLAB Drive/Fichiers_Matlab_sujetB/Fichiers Matlab/STL/EFFECTEUR_Défaut_sldprt.STL  UnitType=Custom  ExtGeomFileUnits=mm  StepReaderType=HEX  ExportConvexHullGeometry=off  InertiaType=Custom  BasedOnType=Density  Density=1000  DensityUnits=kg/(m^3)  Mass=0.013453568991832839  MassUnits=kg  CenterOfMass=[-17.212650388480686 -9.9626588451280398 5.5774208666899616]  CenterOfMassUnits=mm  MomentsOfInertia=[1.2849612996466211 1.3154199043910564 2.2338709867359823]  MomentsOfInertiaUnits=kg*mm^2  ProductsOfInertia=[0.035925388048610812 0.056750034506765974 -0.058662844210309435]  ProductsOfInertiaUnits=kg*mm^2  GraphicType=FromGeometry  MarkerShape=Sphere  MarkerSize=10  GraphicVisPropType=SimpleVisualProperties  GraphicDiffuseColor=[0.792156862745098 0.81960784313725488 0.93333333333333335]  GraphicOpacity=1  GraphicSpecularColor=[0.5 0.5 0.5 1.0]  GraphicAmbientColor=[0.15 0.15 0.15 1.0]  GraphicEmissiveColor=[0.0 0.0 0.0 1.0]  GraphicShininess=75  DoExposeReferenceFrame=on  SerializedFrames=<Frames/>
  F : PMIOPort  Side=Left
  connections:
  Solid/RConn1 -- ReferenceFrame/RConn1 -- F/RConn1

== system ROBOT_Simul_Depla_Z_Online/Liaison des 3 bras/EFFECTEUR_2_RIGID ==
  ReferenceFrame : sm_lib/Frames and Transforms/Reference Frame
  Solid : sm_lib/Body Elements/File Solid  ExtGeomFileName=/MATLAB Drive/Fichiers_Matlab_sujetB/Fichiers Matlab/STL/EFFECTEUR_Défaut_sldprt.STL  UnitType=Custom  ExtGeomFileUnits=mm  StepReaderType=HEX  ExportConvexHullGeometry=off  InertiaType=Custom  BasedOnType=Density  Density=1000  DensityUnits=kg/(m^3)  Mass=0.013453568991832839  MassUnits=kg  CenterOfMass=[-17.212650388480686 -9.9626588451280398 5.5774208666899616]  CenterOfMassUnits=mm  MomentsOfInertia=[1.2849612996466211 1.3154199043910564 2.2338709867359823]  MomentsOfInertiaUnits=kg*mm^2  ProductsOfInertia=[0.035925388048610812 0.056750034506765974 -0.058662844210309435]  ProductsOfInertiaUnits=kg*mm^2  GraphicType=FromGeometry  MarkerShape=Sphere  MarkerSize=10  GraphicVisPropType=SimpleVisualProperties  GraphicDiffuseColor=[0.792156862745098 0.81960784313725488 0.93333333333333335]  GraphicOpacity=1  GraphicSpecularColor=[0.5 0.5 0.5 1.0]  GraphicAmbientColor=[0.15 0.15 0.15 1.0]  GraphicEmissiveColor=[0.0 0.0 0.0 1.0]  GraphicShininess=75  DoExposeReferenceFrame=on  SerializedFrames=<Frames/>
  F : PMIOPort  Side=Left
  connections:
  Solid/RConn1 -- ReferenceFrame/RConn1 -- F/RConn1

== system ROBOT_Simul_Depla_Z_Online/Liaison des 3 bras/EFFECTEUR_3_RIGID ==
  ReferenceFrame : sm_lib/Frames and Transforms/Reference Frame
  Solid : sm_lib/Body Elements/File Solid  ExtGeomFileName=/MATLAB Drive/Fichiers_Matlab_sujetB/Fichiers Matlab/STL/EFFECTEUR_Défaut_sldprt.STL  UnitType=Custom  ExtGeomFileUnits=mm  StepReaderType=HEX  ExportConvexHullGeometry=off  InertiaType=Custom  BasedOnType=Density  Density=1000  DensityUnits=kg/(m^3)  Mass=0.013453568991832839  MassUnits=kg  CenterOfMass=[-17.212650388480686 -9.9626588451280398 5.5774208666899616]  CenterOfMassUnits=mm  MomentsOfInertia=[1.2849612996466211 1.3154199043910564 2.2338709867359823]  MomentsOfInertiaUnits=kg*mm^2  ProductsOfInertia=[0.035925388048610812 0.056750034506765974 -0.058662844210309435]  ProductsOfInertiaUnits=kg*mm^2  GraphicType=FromGeometry  MarkerShape=Sphere  MarkerSize=10  GraphicVisPropType=SimpleVisualProperties  GraphicDiffuseColor=[0.792156862745098 0.81960784313725488 0.93333333333333335]  GraphicOpacity=1  GraphicSpecularColor=[0.5 0.5 0.5 1.0]  GraphicAmbientColor=[0.15 0.15 0.15 1.0]  GraphicEmissiveColor=[0.0 0.0 0.0 1.0]  GraphicShininess=75  DoExposeReferenceFrame=on  SerializedFrames=<Frames/>
  F : PMIOPort  Side=Left
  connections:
  Solid/RConn1 -- ReferenceFrame/RConn1 -- F/RConn1

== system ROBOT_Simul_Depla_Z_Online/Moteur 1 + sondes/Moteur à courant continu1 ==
  note: Kv = 1.18e-1
  Frottement : fl_lib/Mechanical/Rotational Elements/Rotational Friction  brkwy_trq=2.43e-3 N*m  brkwy_vel=0.030296 rad/s  Col_trq=2.43e-3 N*m  visc_coef=2e-6 N*m/(rad/s)  w_specify=off  w_priority=None  w=0 rad/s  w_nominal_specify=off  w_nominal_value=1  w_nominal_unit=rad/s  t_specify=off  t_priority=None  t=0 N*m  t_nominal_specify=off  t_nominal_value=1  t_nominal_unit=N*m
  Inductance induit 35mH : fl_lib/Electrical/Electrical Elements/Inductor  l=35 mH  r=0 Ohm  g=1e-09 1/Ohm  i_specify=off  i_priority=None  i=0 A  i_nominal_specify=off  i_nominal_value=1  i_nominal_unit=A  v_specify=off  v_priority=None  v=0 V  v_nominal_specify=off  v_nominal_value=1  v_nominal_unit=V  i_L_specify=on  i_L_priority=High  i_L=0 A  i_L_nominal_specify=off  i_L_nominal_value=1  i_L_nominal_unit=A
  Inertie Je 10e-6 : fl_lib/Mechanical/Rotational Elements/Inertia  inertia=10.5e-6 kg*m^2  num_ports=foundation.enum.numPorts2.one  w_specify=on  w_priority=High  w=0 rad/s  w_nominal_specify=off  w_nominal_value=1  w_nominal_unit=rad/s  t_specify=off  t_priority=None  t=0 N*m  t_nominal_specify=off  t_nominal_value=1  t_nominal_unit=N*m
  Moteur parfait : fl_lib/Electrical/Electrical Elements/Rotational Electromechanical Converter  K=1.18e-1 V/(rad/s)  i_specify=off  i_priority=None  i=0 A  i_nominal_specify=off  i_nominal_value=1  i_nominal_unit=A  v_specify=off  v_priority=None  v=0 V  v_nominal_specify=off  v_nominal_value=1  v_nominal_unit=V  t_specify=off  t_priority=None  t=0 N*m  t_nominal_specify=off  t_nominal_value=1  t_nominal_unit=N*m  w_specify=off  w_priority=None  w=0 rad/s  w_nominal_specify=off  w_nominal_value=1  w_nominal_unit=rad/s
  Rinduit 38 Ohms : fl_lib/Electrical/Electrical Elements/Resistor  Tag=Factory Generic  R=38 Ohm  i_specify=off  i_priority=None  i=0 A  i_nominal_specify=off  i_nominal_value=1  i_nominal_unit=A  v_specify=off  v_priority=None  v=0 V  v_nominal_specify=off  v_nominal_value=1  v_nominal_unit=V
  V+ : PMIOPort  Side=Left
  R : PMIOPort  Port=2  Side=Right
  C : PMIOPort  Port=3  Side=Right
  V- : PMIOPort  Port=4  Side=Left
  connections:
  C/RConn1 -- Moteur parfait/RConn2 -- Frottement/RConn1
  R/RConn1 -- Inertie Je 10e-6/LConn1 -- Moteur parfait/LConn2 -- Frottement/LConn1
  Inductance induit 35mH/LConn1 -- Rinduit 38 Ohms/RConn1
  Rinduit 38 Ohms/LConn1 -- V+/RConn1
  V-/RConn1 -- Moteur parfait/RConn1
  Moteur parfait/LConn1 -- Inductance induit 35mH/RConn1

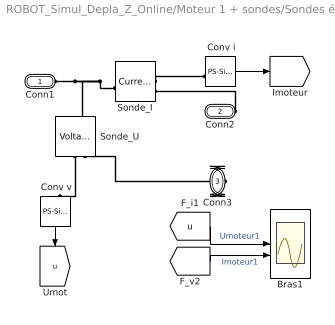
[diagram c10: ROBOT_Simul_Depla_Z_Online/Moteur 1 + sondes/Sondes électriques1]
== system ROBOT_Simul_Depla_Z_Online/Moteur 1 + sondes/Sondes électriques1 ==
  " Conv i" : nesl_utility/PS-Simulink Converter  PhysicalDomain=network_engine_domain  SubClassName=ps_output  LeftPortType=input  RightPortType=output  PseudoPeriodic=off  Frequencies=[]  VectorFormat=1-D array  Unit=1  AffineConversion=off
  " Conv v" : nesl_utility/PS-Simulink Converter  PhysicalDomain=network_engine_domain  SubClassName=ps_output  LeftPortType=input  RightPortType=output  PseudoPeriodic=off  Frequencies=[]  VectorFormat=1-D array  Unit=1  AffineConversion=off
  Bras1 : Scope  NumInputPorts=2
  Sonde_I : fl_lib/Electrical/Electrical Sensors/Current Sensor
  Sonde_U : fl_lib/Electrical/Electrical Sensors/Voltage Sensor
  Conn1 : PMIOPort  Side=Left
  Conn2 : PMIOPort  Port=2  Side=Right
  Conn3 : PMIOPort  Port=3  Side=Right
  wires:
  [i] -> Bras1/2  "Imoteur1"
  [u] -> Bras1/1  "Umoteur1"
  " Conv i"/1 -> [i]
  " Conv v"/1 -> [u]
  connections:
  Conn3/RConn1 -- Sonde_U/RConn2
  Conn2/RConn1 -- Sonde_I/RConn2
  Sonde_I/LConn1 -- Sonde_U/LConn1 -- Conn1/RConn1
  Sonde_U/RConn1 -- " Conv v"/LConn1
  Sonde_I/RConn1 -- " Conv i"/LConn1

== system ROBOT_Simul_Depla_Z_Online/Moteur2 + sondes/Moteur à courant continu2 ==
  note: Kv = 1.18e-1
  Frottement : fl_lib/Mechanical/Rotational Elements/Rotational Friction  brkwy_trq=2.43e-3 N*m  brkwy_vel=0.030296 rad/s  Col_trq=2.43e-3 N*m  visc_coef=2e-6 N*m/(rad/s)  w_specify=off  w_priority=None  w=0 rad/s  w_nominal_specify=off  w_nominal_value=1  w_nominal_unit=rad/s  t_specify=off  t_priority=None  t=0 N*m  t_nominal_specify=off  t_nominal_value=1  t_nominal_unit=N*m
  Inductance induit 35mH : fl_lib/Electrical/Electrical Elements/Inductor  l=35 mH  r=0 Ohm  g=1e-09 1/Ohm  i_specify=off  i_priority=None  i=0 A  i_nominal_specify=off  i_nominal_value=1  i_nominal_unit=A  v_specify=off  v_priority=None  v=0 V  v_nominal_specify=off  v_nominal_value=1  v_nominal_unit=V  i_L_specify=on  i_L_priority=High  i_L=0 A  i_L_nominal_specify=off  i_L_nominal_value=1  i_L_nominal_unit=A
  Inertie Je 10e-6 : fl_lib/Mechanical/Rotational Elements/Inertia  inertia=10.5e-6 kg*m^2  num_ports=foundation.enum.numPorts2.one  w_specify=on  w_priority=High  w=0 rad/s  w_nominal_specify=off  w_nominal_value=1  w_nominal_unit=rad/s  t_specify=off  t_priority=None  t=0 N*m  t_nominal_specify=off  t_nominal_value=1  t_nominal_unit=N*m
  Moteur parfait : fl_lib/Electrical/Electrical Elements/Rotational Electromechanical Converter  K=1.18e-1 V/(rad/s)  i_specify=off  i_priority=None  i=0 A  i_nominal_specify=off  i_nominal_value=1  i_nominal_unit=A  v_specify=off  v_priority=None  v=0 V  v_nominal_specify=off  v_nominal_value=1  v_nominal_unit=V  t_specify=off  t_priority=None  t=0 N*m  t_nominal_specify=off  t_nominal_value=1  t_nominal_unit=N*m  w_specify=off  w_priority=None  w=0 rad/s  w_nominal_specify=off  w_nominal_value=1  w_nominal_unit=rad/s
  Rinduit 38 Ohms : fl_lib/Electrical/Electrical Elements/Resistor  Tag=Factory Generic  R=38 Ohm  i_specify=off  i_priority=None  i=0 A  i_nominal_specify=off  i_nominal_value=1  i_nominal_unit=A  v_specify=off  v_priority=None  v=0 V  v_nominal_specify=off  v_nominal_value=1  v_nominal_unit=V
  V+ : PMIOPort  Side=Left
  R : PMIOPort  Port=2  Side=Right
  C : PMIOPort  Port=3  Side=Right
  V- : PMIOPort  Port=4  Side=Left
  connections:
  Moteur parfait/LConn1 -- Inductance induit 35mH/RConn1
  V-/RConn1 -- Moteur parfait/RConn1
  Rinduit 38 Ohms/LConn1 -- V+/RConn1
  Inductance induit 35mH/LConn1 -- Rinduit 38 Ohms/RConn1
  Frottement/LConn1 -- Moteur parfait/LConn2 -- Inertie Je 10e-6/LConn1 -- R/RConn1
  Frottement/RConn1 -- Moteur parfait/RConn2 -- C/RConn1
